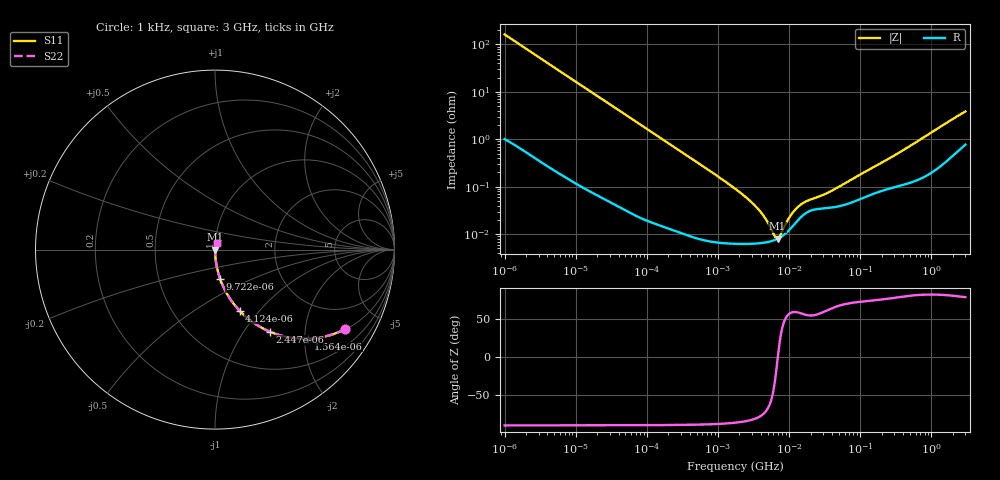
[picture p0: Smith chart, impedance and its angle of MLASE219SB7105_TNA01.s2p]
! MLASE219SB7105_TNA01  S-PARAMETER MODEL  ( Standard Model )
! Model Generated by TAIYO YUDEN Corporation (http://www.ty-top.com)
! Version 1.0
! TAIYO YUDEN Control No. 220601
! Copyright(c) 2009 TAIYO YUDEN CO.,LTD. All Rights Reserved.
! Product Description (link to TY-COMPAS)
! https://ds.yuden.co.jp/TYCOMPAS/or/detail?pn=MLASE219SB7105KTNA01&u=M
! Products Name : Multilayer Ceramic Capacitors
! Characteristics :
!  Capacitance : 1 [uF] , Rated Voltage : 16 [V] , TCC : X7R
!  Case Size : 2.0 x 1.25 / 0.079 x 0.049 [mm/inch] , Thickness : 0.85 / 0.033 [mm/inch]
!  (Conditions: Temperature = 25 [degC] , DC Bias Voltage = 0 [V])
! External Node Assignments :
!  1  o---| |---o  2
! GND o---------o GND
! Frequency Range : 1kHz  -  3GHz  [ 401 STEP ]
# MHZ S RI R 50
! Freq[MHz].  S11 Real  S11 Imag  S21 Real  S21 Imag  S12 Real  S12 Imag  S22 Real  S22 Imag
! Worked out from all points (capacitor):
!   401 points, 1 kHz to 3 GHz, reference 50 ohm
!   read as one part in series: C = 980 nF near 1.077 kHz
!   lowest |Z| = 8.01 mohm at 6.882 MHz (marker M1)
!   series resonance near 6.926 MHz, so ESL is about 540 pH
!   S11 on the Smith chart (normalised r, x): 1 kHz: 1.02, -3.24; 1.564 kHz: 1.01, -2.08; 2.447 kHz: 1.01, -1.33; 4.124 kHz: 1.01, -0.79; 9.722 kHz: 1.00, -0.34; 3 GHz: 1.02, +0.08
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0.001  0.7231 -0.4444  0.2769 0.4444  0.2769 0.4444  0.7231 -0.4444
0.001564  0.5187 -0.4964  0.4813 0.4964  0.4813 0.4964  0.5187 -0.4964
0.002447  0.3079 -0.4584  0.6921 0.4584  0.6921 0.4584  0.3079 -0.4584
0.004124  0.1369 -0.3405  0.8631 0.3405  0.8631 0.3405  0.1369 -0.3405
0.005988  0.0708 -0.253  0.9292 0.253  0.9292 0.253  0.0708 -0.253
0.009722  0.0287 -0.1633  0.9713 0.1633  0.9713 0.1633  0.0287 -0.1633
0.01216  0.0188 -0.1321  0.9812 0.1321  0.9812 0.1321  0.0188 -0.1321
0.033275  0.00288 -0.0493  0.9971 0.0493  0.9971 0.0493  0.00288 -0.0493
0.147855  0.00028 -0.0112  0.9997 0.0112  0.9997 0.0112  0.00028 -0.0112
1.732051  6.34e-05 -0.00091  0.9999 0.00091  0.9999 0.00091  6.34e-05 -0.00091
3.517417  6.38e-05 -0.000358  0.9999 0.000358  0.9999 0.000358  6.38e-05 -0.000358
4.566395  6.66e-05 -0.000211  0.9999 0.000211  0.9999 0.000211  6.66e-05 -0.000211
5.928204  7.31e-05 -7.76e-05  0.9999 7.76e-05  0.9999 7.76e-05  7.31e-05 -7.76e-05
6.881678  8.01e-05 -3.16e-06  0.9999 3.16e-06  0.9999 3.16e-06  8.01e-05 -3.16e-06
7.696136  8.8e-05 5.29e-05  0.9999 -5.29e-05  0.9999 -5.29e-05  8.8e-05 5.29e-05
9.991309  0.000122 0.000185  0.9999 -0.000185  0.9999 -0.000185  0.000122 0.000185
12.49624  0.000177 0.000293  0.9998 -0.000293  0.9998 -0.000293  0.000177 0.000293
15.62917  0.00025 0.000376  0.9997 -0.000376  0.9997 -0.000376  0.00025 0.000376
21.06097  0.000321 0.00045  0.9997 -0.00045  0.9997 -0.00045  0.000321 0.00045
39.69685  0.000364 0.000739  0.9996 -0.000739  0.9996 -0.000739  0.000364 0.000739
256.0921  0.000925 0.00385  0.9991 -0.00385  0.9991 -0.00385  0.000925 0.00385
3000  0.00905 0.0372  0.991 -0.0372  0.991 -0.0372  0.00905 0.0372
